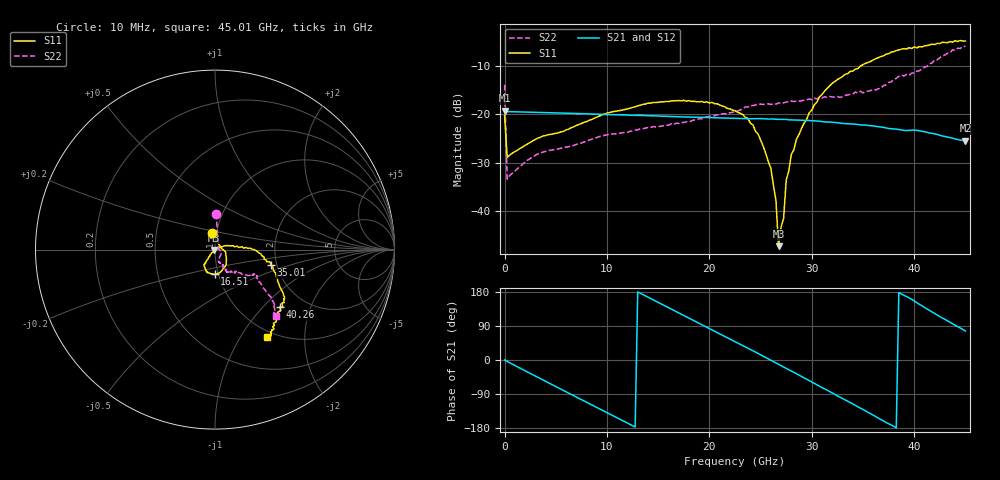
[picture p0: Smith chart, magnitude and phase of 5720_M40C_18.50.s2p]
! Device:  ADRF5720
! Description: 0.5dB LSB GaAs MMIC 6-bit Digital Attenuator
! Frequency:  0.000009 -  40 GHz
! Ports:
!	RF1	= Port 1
!	RF2	= Port 2
! Vdd:  3.3 Volt
! Vss:  -3.3 Volt
! Control:  0/3.3 Volt
! State:  18.50 dB attenuation
! Data:  The device was measured using G-S-G Probes on a matrix board.
!  Data was collected using an calibrated 4 port network analyzer.
!  The reference plane for this measurement is at the launchers.
! Note:  Analog Devices supplies this data as a sample of measured data
!  for this product.  Your particular data for this product may vary.
!  Data was taken at -40 degrees C.
!  Analog Devices reserves the right to change this data at anytime.
# GHZ S DB R 45.0
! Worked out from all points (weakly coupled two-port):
!   181 points, 10 MHz to 45.01 GHz, reference 45 ohm
!   highest |S21| = -19.30 dB at 10 MHz (marker M1); lowest = -25.5 dB at 45.01 GHz (marker M2)
!   lowest |S11| = -47.3 dB at 26.76 GHz (marker M3), VSWR 1.01, Z = 44.7 - j0.214 ohm
!   |S11| at or under -10 dB: start of sweep to 34.82 GHz
!   |S22| runs from -33.4 to -6.0 dB; largest |S21 - S12| = 0.00041
!   S11 on the Smith chart (normalised r, x): 10 MHz: 0.95, +0.18; 16.51 GHz: 0.96, -0.27; 35.01 GHz: 1.86, -0.36; 40.26 GHz: 1.50, -1.26; 45.01 GHz: 0.91, -1.32
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0.01  -20.29 101.6  -19.30 0.2  -19.32 0.2  -13.95 88.2
0.26  -28.94 14.8  -19.48 -3.8  -19.50 -3.9  -33.42 22.3
3.26  -24.95 -9.5  -19.65 -45.8  -19.67 -45.9  -28.20 -28.5
7.76  -21.69 -39.3  -19.92 -108.0  -19.94 -108.0  -25.76 -61.7
15.26  -17.48 -83.0  -20.40 148.4  -20.42 148.4  -22.51 -71.5
16.51  -17.26 -90.7  -20.52 131.2  -20.54 131.2  -22.16 -69.5
20.26  -17.57 -110.5  -20.73 79.4  -20.75 79.3  -20.40 -63.8
22.76  -19.58 -125.7  -20.88 44.9  -20.90 44.9  -19.35 -64.2
24.26  -22.23 -126.9  -20.95 24.4  -20.97 24.3  -18.24 -62.7
26.01  -31.16 -133.4  -21.01 -0.5  -21.03 -0.6  -18.01 -62.1
26.51  -37.88 -125.7  -21.05 -7.9  -21.07 -8.0  -17.93 -63.2
26.76  -47.28 -146.3  -21.09 -11.3  -21.11 -11.4  -17.69 -61.2
27.01  -43.32 -24.4  -21.09 -14.7  -21.12 -14.8  -17.71 -62.9
27.26  -41.51 36.9  -21.10 -18.4  -21.12 -18.5  -17.68 -61.2
27.51  -33.63 14.5  -21.09 -22.1  -21.11 -22.2  -17.49 -62.4
28.01  -28.32 19.6  -21.19 -29.0  -21.21 -29.2  -17.31 -62.8
30.26  -18.05 8.9  -21.39 -61.6  -21.41 -61.8  -16.69 -61.0
32.01  -13.63 0.4  -21.69 -87.1  -21.71 -87.2  -16.44 -56.1
35.01  -9.78 -15.5  -22.25 -130.5  -22.27 -130.6  -15.61 -47.0
37.76  -7.18 -31.5  -23.01 -171.5  -23.03 -171.7  -13.35 -40.8
40.26  -6.32 -41.5  -23.34 151.5  -23.37 151.3  -11.14 -31.7
45.01  -4.89 -59.2  -25.50 76.6  -25.52 76.5  -5.98 -47.2
